(* Logix 5000 AddOnInstructionDefinition export EipIoDataMapping_PAL_EIP; software revision 37.00; part 2 of 2 *)
(* tags used below, declared in another part *)
   mod_EipOutputData : _054B:PAL_EIP_3E1CE89C:O:0;   // Module defined using SINT data type
   ref_InstanceOfPal : PneumaticAutomationLink_UDT;   // Reference to an instance of the PneumaticAutomationLink_UDT
(* EipIoDataMapping_PAL_EIP, continued *)

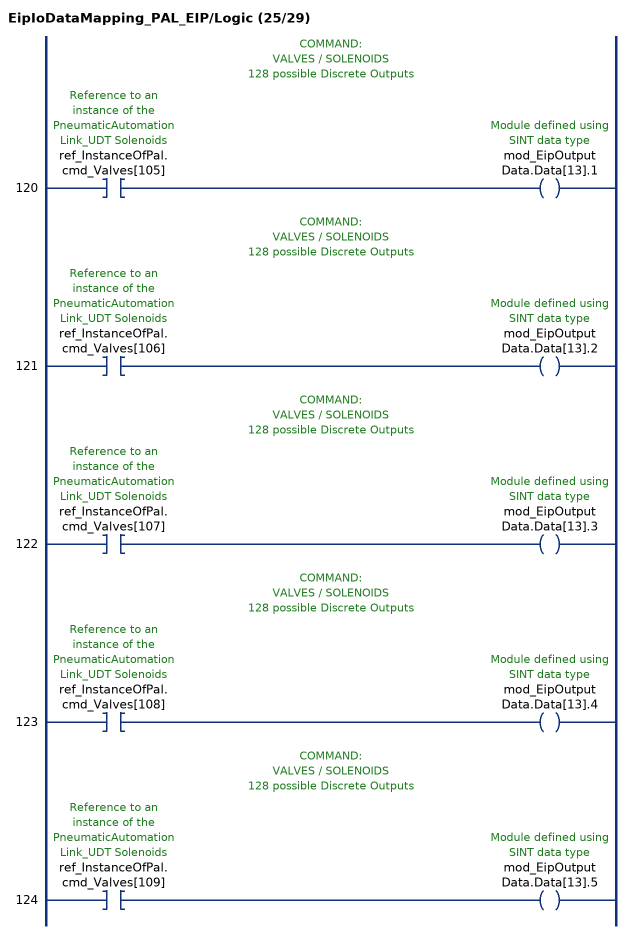
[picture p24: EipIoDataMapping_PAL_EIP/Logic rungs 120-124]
   // COMMAND:
   // VALVES / SOLENOIDS
   // 128 possible Discrete Outputs
   120: XIC(ref_InstanceOfPal.cmd_Valves[105])OTE(mod_EipOutputData.Data[13].1);
   // COMMAND:
   // VALVES / SOLENOIDS
   // 128 possible Discrete Outputs
   121: XIC(ref_InstanceOfPal.cmd_Valves[106])OTE(mod_EipOutputData.Data[13].2);
   // COMMAND:
   // VALVES / SOLENOIDS
   // 128 possible Discrete Outputs
   122: XIC(ref_InstanceOfPal.cmd_Valves[107])OTE(mod_EipOutputData.Data[13].3);
   // COMMAND:
   // VALVES / SOLENOIDS
   // 128 possible Discrete Outputs
   123: XIC(ref_InstanceOfPal.cmd_Valves[108])OTE(mod_EipOutputData.Data[13].4);
   // COMMAND:
   // VALVES / SOLENOIDS
   // 128 possible Discrete Outputs
   124: XIC(ref_InstanceOfPal.cmd_Valves[109])OTE(mod_EipOutputData.Data[13].5);
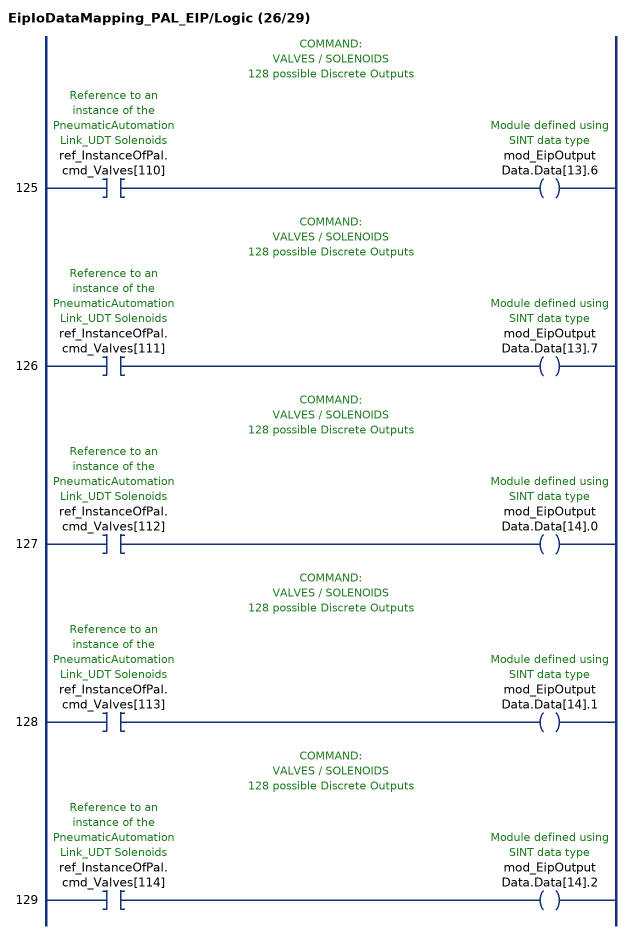
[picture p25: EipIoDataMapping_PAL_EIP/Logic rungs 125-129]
   // COMMAND:
   // VALVES / SOLENOIDS
   // 128 possible Discrete Outputs
   125: XIC(ref_InstanceOfPal.cmd_Valves[110])OTE(mod_EipOutputData.Data[13].6);
   // COMMAND:
   // VALVES / SOLENOIDS
   // 128 possible Discrete Outputs
   126: XIC(ref_InstanceOfPal.cmd_Valves[111])OTE(mod_EipOutputData.Data[13].7);
   // COMMAND:
   // VALVES / SOLENOIDS
   // 128 possible Discrete Outputs
   127: XIC(ref_InstanceOfPal.cmd_Valves[112])OTE(mod_EipOutputData.Data[14].0);
   // COMMAND:
   // VALVES / SOLENOIDS
   // 128 possible Discrete Outputs
   128: XIC(ref_InstanceOfPal.cmd_Valves[113])OTE(mod_EipOutputData.Data[14].1);
   // COMMAND:
   // VALVES / SOLENOIDS
   // 128 possible Discrete Outputs
   129: XIC(ref_InstanceOfPal.cmd_Valves[114])OTE(mod_EipOutputData.Data[14].2);
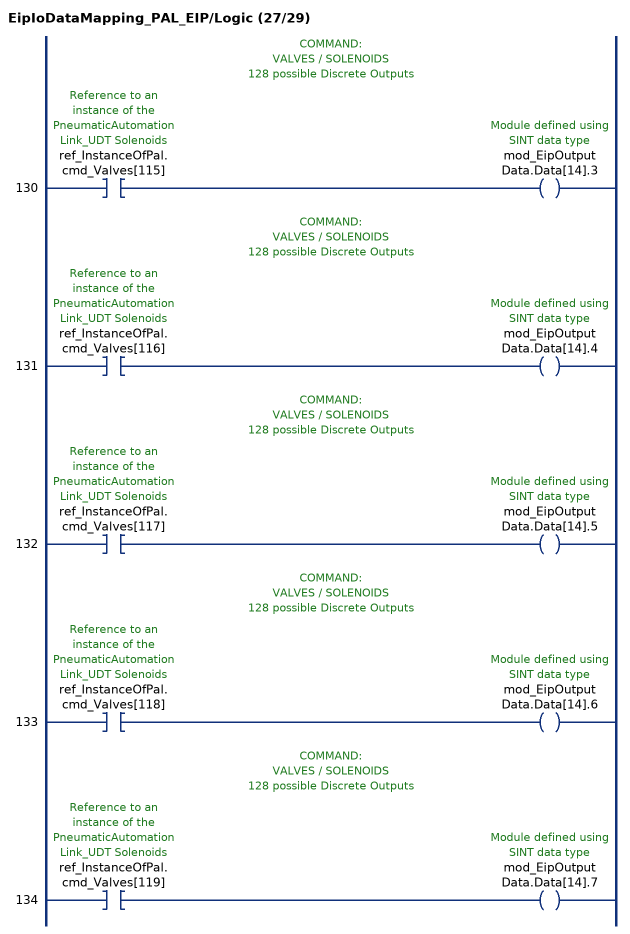
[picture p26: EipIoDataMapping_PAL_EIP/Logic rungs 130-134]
   // COMMAND:
   // VALVES / SOLENOIDS
   // 128 possible Discrete Outputs
   130: XIC(ref_InstanceOfPal.cmd_Valves[115])OTE(mod_EipOutputData.Data[14].3);
   // COMMAND:
   // VALVES / SOLENOIDS
   // 128 possible Discrete Outputs
   131: XIC(ref_InstanceOfPal.cmd_Valves[116])OTE(mod_EipOutputData.Data[14].4);
   // COMMAND:
   // VALVES / SOLENOIDS
   // 128 possible Discrete Outputs
   132: XIC(ref_InstanceOfPal.cmd_Valves[117])OTE(mod_EipOutputData.Data[14].5);
   // COMMAND:
   // VALVES / SOLENOIDS
   // 128 possible Discrete Outputs
   133: XIC(ref_InstanceOfPal.cmd_Valves[118])OTE(mod_EipOutputData.Data[14].6);
   // COMMAND:
   // VALVES / SOLENOIDS
   // 128 possible Discrete Outputs
   134: XIC(ref_InstanceOfPal.cmd_Valves[119])OTE(mod_EipOutputData.Data[14].7);
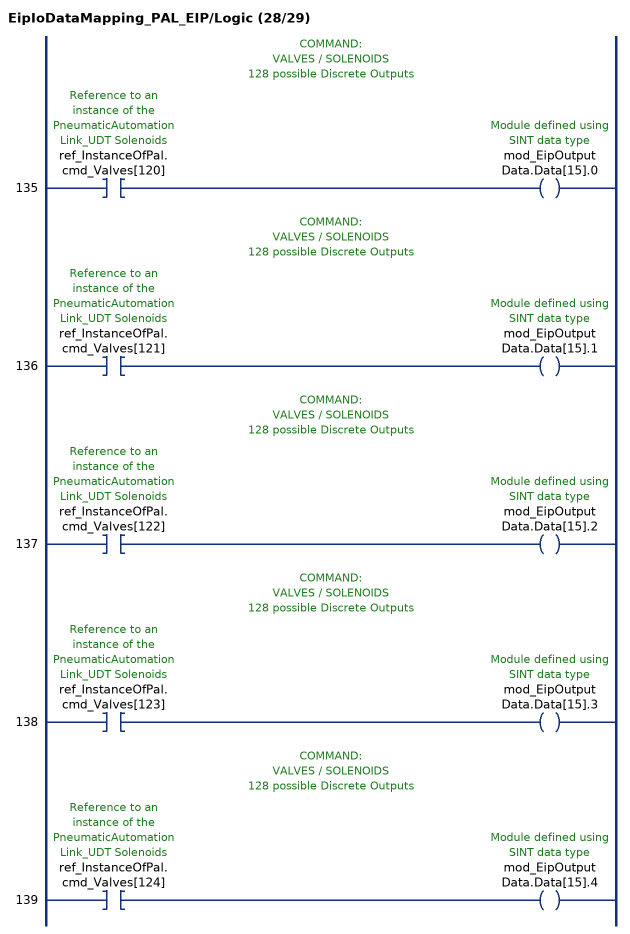
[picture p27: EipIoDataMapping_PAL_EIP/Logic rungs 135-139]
   // COMMAND:
   // VALVES / SOLENOIDS
   // 128 possible Discrete Outputs
   135: XIC(ref_InstanceOfPal.cmd_Valves[120])OTE(mod_EipOutputData.Data[15].0);
   // COMMAND:
   // VALVES / SOLENOIDS
   // 128 possible Discrete Outputs
   136: XIC(ref_InstanceOfPal.cmd_Valves[121])OTE(mod_EipOutputData.Data[15].1);
   // COMMAND:
   // VALVES / SOLENOIDS
   // 128 possible Discrete Outputs
   137: XIC(ref_InstanceOfPal.cmd_Valves[122])OTE(mod_EipOutputData.Data[15].2);
   // COMMAND:
   // VALVES / SOLENOIDS
   // 128 possible Discrete Outputs
   138: XIC(ref_InstanceOfPal.cmd_Valves[123])OTE(mod_EipOutputData.Data[15].3);
   // COMMAND:
   // VALVES / SOLENOIDS
   // 128 possible Discrete Outputs
   139: XIC(ref_InstanceOfPal.cmd_Valves[124])OTE(mod_EipOutputData.Data[15].4);
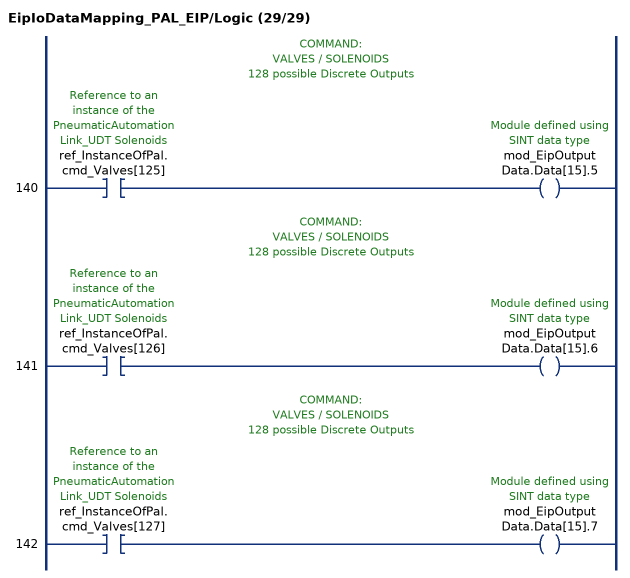
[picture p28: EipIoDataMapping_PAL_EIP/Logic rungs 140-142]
   // COMMAND:
   // VALVES / SOLENOIDS
   // 128 possible Discrete Outputs
   140: XIC(ref_InstanceOfPal.cmd_Valves[125])OTE(mod_EipOutputData.Data[15].5);
   // COMMAND:
   // VALVES / SOLENOIDS
   // 128 possible Discrete Outputs
   141: XIC(ref_InstanceOfPal.cmd_Valves[126])OTE(mod_EipOutputData.Data[15].6);
   // COMMAND:
   // VALVES / SOLENOIDS
   // 128 possible Discrete Outputs
   142: XIC(ref_InstanceOfPal.cmd_Valves[127])OTE(mod_EipOutputData.Data[15].7);
END_ROUTINE
END_ADD_ON_INSTRUCTION
